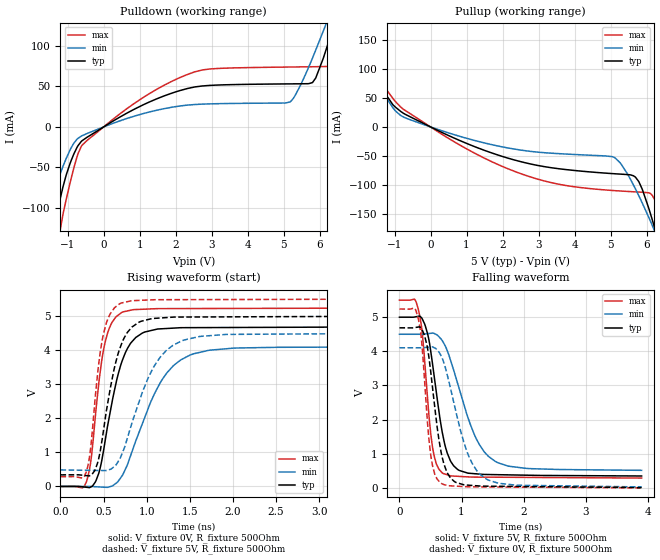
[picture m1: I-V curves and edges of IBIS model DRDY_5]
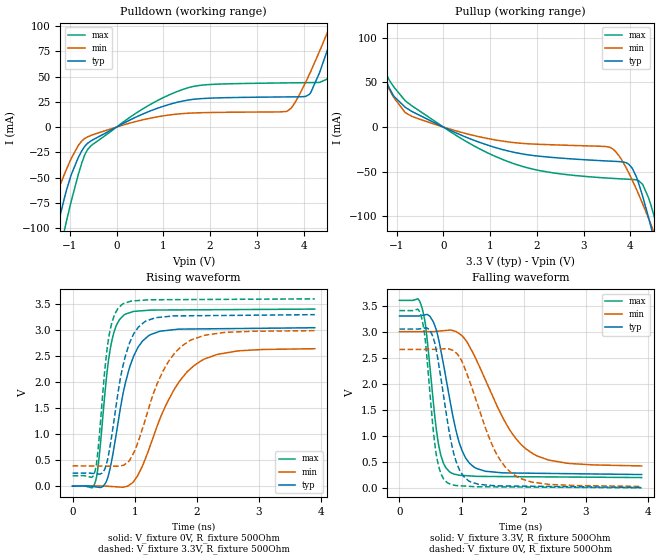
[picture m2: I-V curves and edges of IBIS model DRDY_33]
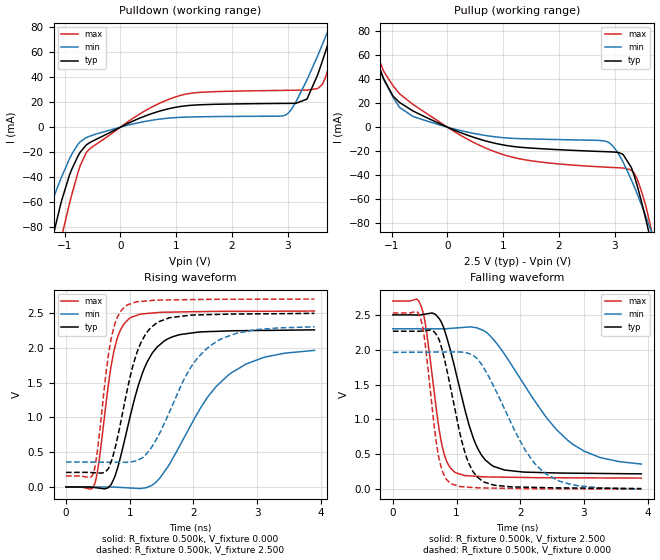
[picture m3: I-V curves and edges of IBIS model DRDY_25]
| Texas Instruments Incorporated
| Marketing part#   Voltage Range   Package-type   #pins/pkg drawing
| ADS1220PW   2.3V - 5.5V   TSSOP   16/PW
| ADS1220RVA   2.3V - 5.5V   QFN   16/RVA
| ADS1120PW   2.3V - 5.5V   TSSOP   16/PW
| ADS1120RVA   2.3V - 5.5V   QFN   16/RVA
[IBIS Ver]   4.0
[File name]   ads1220.ibs
[File Rev]   1.1
[Date]   1/15/2014
[Source]   Model built from TISpice simulations at:
   Texas Instruments Incorporated.
   Webench Design Center
   12500 TI Blvd
   Dallas, TX -75243
   For Support e-mail: elab_ibis@list.ti.com
[Notes]   Revision History
   1.1: 01/15/2014
   - Add device ADS1120PW and ADS1120RVA to supported devices
   and change name of components to represent both devices with 'x.'
   1.0   | Initial Release
   - C_comp although listed in numerical order of value are
   obtained from varying PVT conditions. For PVT conditions
   for each specific value refer the buffer description under
   respective [Model]. IBIS model user is responsible for using
   appropriate C_comp to simulate for Signal Integrity.
[Disclaimer]  This model is designed as an aid for customers of Texas Instruments
 TI and its licensors and suppliers make no warranties, either expressed
 or implied, with respect to this  model, including the warranties of
 merchantability or fitness for a particular purpose.
 The model is provided solely on an "as is" basis. The entire risk as to
 its quality and performance is with the customer.
[Copyright] (C)Copyright 2014 Texas Instruments Incorporated.
   All rights reserved.
[Component]  ADS1x20PW
[Manufacturer]  Texas Instruments
[Package]
|   typ   min   max
R_pkg   0   0   0
L_pkg   0   0   0
C_pkg   0   0   0
[Pin]   signal_name   model_name   R_pin   L_pin   C_pin
1   CLK   DIN   0.19322  2.91462n  0.47845p
2   DGND   GND   0.19290  2.48827n  0.48118p
3   AVSS   GND   0.16877  1.95590n  0.35342p
4   AIN3   TERM   0.16849  1.94998n  0.36106p
5   AIN2   TERM   0.06398  1.50548n  0.40584p
6   REFN0   TERM   0.16819  1.95272n  0.35310p
7   REFP0   TERM   0.20145  2.55201n  0.48267p
8   AIN1   TERM   0.19504  2.93239n  0.47960p
9   AIN0   TERM   0.19504  2.93239n  0.47958p
10   AVDD   POWER   0.20145  2.55201n  0.48241p
11   DVDD   POWER   0.17165  1.97913n  0.35356p
12   DRDY   DRDY   0.09379  1.65190n  0.39123p
13   DOUT   DOUT   0.16644  1.93419n  0.36060p
14   DIN   DIN   0.16865  1.95507n  0.35303p
15   SCLK   DIN   0.19362  2.49377n  0.48147p
16   CS   DIN   0.19322  2.91462n  0.47846p
[Component]  ADS1x20RVA
[Manufacturer]  Texas Instruments
[Package]
|   typ   min   max
R_pkg   0   0   0
L_pkg   0   0   0
C_pkg   0   0   0
[Pin]   signal_name   model_name   R_pin   L_pin   C_pin
1   CLK   DIN   0.06026  0.73141n  0.13625pF
2   DGND   GND   0.06340  0.77403n  0.15300pF
3   AVSS   GND   0.02077  0.40544n  0.18775pF
4   AIN3   TERM   0.06028  0.73169n  0.13612pF
5   AIN2   TERM   0.06127  0.74279n  0.13670pF
6   REFN0   TERM   0.06032  0.72840n  0.14946pF
7   REFP0   TERM   0.06032  0.72772n  0.14944pF
8   AIN1   TERM   0.06127  0.74046n  0.13654pF
9   AIN0   TERM   0.06051  0.72727n  0.13563pF
10   AVDD   POWER   0.03224  0.51093n  0.17648pF
11   DVDD   POWER   0.06123  0.73664n  0.15089pF
12   DRDY   DRDY   0.06048  0.72677n  0.13587pF
13   DOUT   DOUT   0.06057  0.73159n  0.13595pF
14   DIN   DIN   0.06026  0.72711n  0.14916pF
15   SCLK   DIN   0.06026  0.72728n  0.14916pF
16   CS   DIN   0.06037  0.72972n  0.13575pF
[Model Selector]  DIN
DIN_5   5.0V non-modeled pin
DIN_33   3.3V non-modeled pin
DIN_25   2.5V non-modeled pin
[Model Selector]  DRDY
DRDY_5   5.0V non-modeled pin
DRDY_33   3.3V non-modeled pin
DRDY_25   2.5V non-modeled pin
[Model Selector]  DOUT
DOUT_5   5.0V non-modeled pin
DOUT_33   3.3V non-modeled pin
DOUT_25   2.5V non-modeled pin
[Model Selector]  TERM
TERM_5   5.0V non-modeled pin
TERM_33   3.3V non-modeled pin
TERM_25   2.5V non-modeled pin
|   TERM Model
[Model] TERM_33
Model_type Terminator
C_comp   1e-20   1e-20   1e-20
| variable   typ   min   max
[Voltage Range]   3.3V   3.15V   3.45V
[POWER Clamp Reference]  3.3V   3.15V   3.45V
|Operating Temperature
[Temperature Range]   27   125   -40
[Model] TERM_25
Model_type Terminator
C_comp   1e-20   1e-20   1e-20
| variable   typ   min   max
[Voltage Range]   2.5V   2.375V   2.625V
[POWER Clamp Reference]  2.5V   2.375V   2.625V
[GND Clamp Reference]   0.0V   0.0V   0.0V
|Operating Temperature
[Temperature Range]   27   125   -40
[Model] TERM_5
Model_type Terminator
C_comp   1e-20   1e-20   1e-20
| variable   typ   min   max
[Voltage Range]   5.0V   4.5V   5.5V
[POWER Clamp Reference]  5.0V   4.5V   5.5V
[GND Clamp Reference]   0.0V   0.0V   0.0V
|Operating Temperature
[Temperature Range]   27   125   -40
| Models and submodels in the file (12): DRDY_5 (Output), DRDY_33 (Output), DRDY_25 (Output), DOUT_5 (3-state), DOUT_33 (3-state), DOUT_25 (3-state), DIN_5 (Input), DIN_33 (Input), DIN_25 (Input), TERM_33 (Terminator), TERM_25 (Terminator), TERM_5 (Terminator)
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|   DRDY_5 Model
[Model]   DRDY_5
Model_type   Output
Polarity   Non-Inverting
Vmeas = 2.5
Vref = 2.5
Cref = 15pF
Rref = 500
|   typ   min   max
|   (nom PVT)   (Fast PVT)   (slow PVT)
C_comp   2.792p   2.372p   3.227p
|C_comp (ON state)   2.957p   2.508p   3.404p
|C_comp (OFF state)   2.792p   2.372p   3.227p
| Where   nom PVT is  Nominal Process, 5V, 27C
|   Fast PVT is Strong Process, 5.5V, -40C
|   Slow PVT is Weak Process, 4.5V, 125C
[Voltage Range]   5   4.5   5.5
[Temperature Range]   27   125   -40
[Pullup Reference]   5   4.5   5.5
[Pulldown Reference]   0   0   0
[Power Clamp Reference]   5   4.5   5.5
[GND Clamp Reference]   0   0   0
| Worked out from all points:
|   slope of the pulldown table from 0 to 0.75 V, typ, clamps not added: 38.5 ohm
|   slope of the pullup table from 0 to 0.75 V, typ, clamps not added: 34.6 ohm
|   falling waveform, V_fixture 5V, R_fixture 500Ohm: 20-80 % time 231ps typ, 445ps min, 150ps max; typ from 5 V to 0.349 V
|   rising waveform, V_fixture 0V, R_fixture 500Ohm: 20-80 % time 233ps typ, 416ps min, 148ps max; typ from 0 V to 4.68 V
|   rising waveform, V_fixture 5V, R_fixture 500Ohm: 20-80 % time 214ps typ, 369ps min, 139ps max; typ from 0.34 V to 5 V
|   falling waveform, V_fixture 0V, R_fixture 500Ohm: 20-80 % time 203ps typ, 366ps min, 136ps max; typ from 4.69 V to 0.009 V
[Pulldown]
|   Voltage   I(typ)   I(min)   I(max)
-5V       -984.7mA   -666.3mA   -1.34A
-1.835V   -225.5mA   -142.5mA   -320.3mA
-1.52V    -154.3mA   -97.92mA   -220.6mA
-1.25V    -96.93mA   -62.99mA   -138.7mA
-605mV    -17.19mA   -11mA      -22.85mA
2.32V     47.36mA    26.92mA    64.68mA
5.17V     53.16mA    30.73mA    73.97mA
5.8V      54.77mA    84.97mA    74.32mA
6.25V     105.4mA    135.3mA    74.76mA
6.415V    129.1mA    154.2mA    79.06mA
7.09V     229.8mA    232.8mA    195.3mA
10V       695.5mA    589.2mA    793.5mA
[Pullup]
|   Voltage   I(typ)   I(min)   I(max)
-5V       615.3mA    484.3mA    781.6mA
-2.36V    216.2mA    176.1mA    268.1mA
-2.195V   191.6mA    157.1mA    236.3mA
-1.97V    158.2mA    131.4mA    193.3mA
-965mV    33.47mA    26.93mA    42.93mA
820mV     -23.56mA   -16.29mA   -31.34mA
2.95V     -65.85mA   -43.15mA   -89.22mA
5.095V    -80.35mA   -52.09mA   -109.3mA
5.695V    -86.53mA   -106.8mA   -111.6mA
6.25V     -178.5mA   -182.4mA   -127.7mA
6.49V     -231.1mA   -218.4mA   -172.3mA
10V       -1.077A    -812.1mA   -1.299A
[Ramp]
R_load = 500
|   typ   min   max
dV/dt_r   2.81122/2.31953e-10   2.45779/4.13764e-10   3.14302/1.47295e-10
dV/dt_f   2.79077/2.30674e-10   2.39144/4.43892e-10   3.12731/1.49622e-10
[Falling Waveform]
V_fixture = 5V
V_fixture_min = 4.5V
V_fixture_max = 5.5V
R_fixture = 500Ohm
C_fixture = 0F
|   Time   V(typ)   V(min)   V(max)
0s        5V         4.5V       5.5V
301.3ps   5.024V     4.5V       5.249V
371.3ps   4.936V     4.502V     4.473V
529ps     3.685V     4.532V     1.238V
685.9ps   1.663V     4.323V     444.6mV
769.3ps   1.022V     4.02V      383.9mV
935.2ps   542.4mV    3.072V     340.2mV
1.236ns   412mV      1.445V     316.7mV
1.544ns   388.3mV    775.6mV    313.3mV
3.9ns     348.7mV    514.3mV    287.8mV
[Rising Waveform]
V_fixture = 0V
V_fixture_min = 0V
V_fixture_max = 0V
R_fixture = 500Ohm
C_fixture = 0F
|   Time   V(typ)   V(min)   V(max)
0s        4.594nV    7.392nV    3.899nV
301.3ps   -24.2mV    1.124mV    139.9mV
356.5ps   -8.175mV   -908.9uV   823.3mV
413.5ps   178.3mV    -9.035mV   2.296V
505.6ps   1.141V     -22.14mV   4.09V
706.2ps   3.619V     283.1mV    5.102V
873.5ps   4.375V     1.338V     5.194V
1.154ns   4.626V     3.031V     5.221V
1.5ns     4.662V     3.854V     5.223V
3.9ns     4.685V     4.096V     5.238V
[Rising Waveform]
V_fixture = 5V
V_fixture_min = 4.5V
V_fixture_max = 5.5V
R_fixture = 500Ohm
C_fixture = 0F
|   Time   V(typ)   V(min)   V(max)
0s        340.2mV    485.1mV    286.7mV
297.8ps   318.2mV    474.7mV    416.5mV
347ps     325.1mV    472.9mV    1.061V
404.3ps   504.9mV    470.9mV    2.651V
490.1ps   1.488V     467.9mV    4.375V
685.9ps   4.033V     801.1mV    5.363V
829.5ps   4.681V     1.868V     5.454V
1.064ns   4.93V      3.427V     5.479V
1.397ns   4.974V     4.265V     5.485V
3.9ns     4.998V     4.494V     5.5V
[Falling Waveform]
|Gnd
V_fixture = 0V
V_fixture_min = 0V
V_fixture_max = 0V
R_fixture = 500Ohm
C_fixture = 0F
|   Time   V(typ)   V(min)   V(max)
0s        4.688V     4.104V     5.239V
297.8ps   4.711V     4.103V     4.998V
362.6ps   4.642V     4.106V     4.19V
499.9ps   3.458V     4.126V     1.018V
565.1ps   2.423V     4.1V       425.1mV
658.7ps   1.172V     3.912V     150.9mV
819ps     296.5mV    2.942V     59.86mV
1.091ns   81.82mV    1.045V     34.35mV
1.397ns   50.88mV    262.5mV    28.41mV
3.9ns     8.998mV    28.15mV    1.283mV
|   DRDY_33 Model
[Model]   DRDY_33
Model_type   Output
Polarity   Non-Inverting
Vmeas = 1.65
Vref = 1.65
Cref = 15pF
Rref = 500
|   typ   min   max
|   (nom PVT)   (Fast PVT)   (slow PVT)
C_comp   3.004p   2.545p   3.470p
|C_comp (ON state)   3.156p   2.689p   3.615p
|C_comp (OFF state)   3.004p   2.545p   3.470p
| Where   nom PVT is  Nominal Process, 3.3V, 27C
|   Fast PVT is Strong Process, 3.6V, -40C
|   Slow PVT is Weak Process, 3.0V, 125C
[Voltage Range]   3.3   3   3.6
[Temperature Range]   27   125   -40
[Pullup Reference]   3.3   3   3.6
[Pulldown Reference]   0   0   0
[Power Clamp Reference]   3.3   3   3.6
[GND Clamp Reference]   0   0   0
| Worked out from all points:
|   slope of the pulldown table from 0 to 0.495 V, typ, clamps not added: 42.9 ohm
|   slope of the pullup table from 0 to 0.495 V, typ, clamps not added: 42.9 ohm
|   falling waveform, V_fixture 3.3V, R_fixture 500Ohm: 20-80 % time 306ps typ, 654ps min, 183ps max; typ from 3.3 V to 0.256 V
|   rising waveform, V_fixture 0V, R_fixture 500Ohm: 20-80 % time 316ps typ, 614ps min, 182ps max; typ from 0 V to 3.04 V
|   rising waveform, V_fixture 3.3V, R_fixture 500Ohm: 20-80 % time 283ps typ, 517ps min, 168ps max; typ from 0.248 V to 3.3 V
|   falling waveform, V_fixture 0V, R_fixture 500Ohm: 20-80 % time 261ps typ, 507ps min, 163ps max; typ from 3.05 V to 0.008 V
[Pulldown]
|   Voltage   I(typ)   I(min)   I(max)
-3.3V     -573.5mA   -376.1mA   -791.3mA
-1.736V   -202.6mA   -128mA     -288.6mA
-1.3V     -106.7mA   -68.95mA   -152.7mA
-1.112V   -69.7mA    -46.43mA   -101.8mA
-617.1mV  -16mA      -9.682mA   -22.14mA
709.5mV   15.75mA    8.689mA    22.07mA
1.68V     27.68mA    14.03mA    40.59mA
3.64V     29.87mA    15.63mA    43.78mA
4.135V    32.91mA    53.13mA    44.04mA
4.561V    83.38mA    99.24mA    52.5mA
4.957V    140.9mA    144.3mA    119.8mA
6.6V      389.2mA    336mA      438.2mA
[Pullup]
|   Voltage   I(typ)   I(min)   I(max)
-3.3V     357.5mA    285.1mA    450.1mA
-1.934V   152.6mA    127mA      186.1mA
-1.399V   75.08mA    67.22mA    86.57mA
-1.053V   34.09mA    32.4mA     44.39mA
-636.9mV  16.5mA     11.25mA    22.48mA
1.403V    -27.01mA   -16.73mA   -39.08mA
3.571V    -38.19mA   -22.89mA   -57.36mA
4.046V    -46.68mA   -60.1mA    -58.74mA
4.264V    -77.65mA   -86.15mA   -64.23mA
4.442V    -112mA     -109.4mA   -87.85mA
4.58V     -141mA     -128.5mA   -116mA
6.6V      -616.6mA   -451.2mA   -757.4mA
[Ramp]
R_load = 500
|   typ   min   max
dV/dt_r   1.82672/3.14339e-10   1.58478/6.10418e-10   2.04187/1.81599e-10
dV/dt_f   1.82616/3.05643e-10   1.54681/6.52787e-10   2.04071/1.8322e-10
[Falling Waveform]
V_fixture = 3.3V
V_fixture_min = 3V
V_fixture_max = 3.6V
R_fixture = 500Ohm
C_fixture = 0F
|   Time   V(typ)   V(min)   V(max)
0s        3.3V       3V         3.6V
357.9ps   3.31V      3V         3.479V
431ps     3.327V     3V         3.017V
622.4ps   2.897V     3.008V     885.9mV
804.8ps   1.736V     3.028V     311.6mV
960.8ps   877.3mV    2.962V     244mV
1.128ns   474.3mV    2.715V     230.9mV
1.664ns   288.6mV    1.348V     217.5mV
2.039ns   283.1mV    746.2mV    214.4mV
3.9ns     256.4mV    422mV      198.8mV
[Rising Waveform]
V_fixture = 0V
V_fixture_min = 0V
V_fixture_max = 0V
R_fixture = 500Ohm
C_fixture = 0F
|   Time   V(typ)   V(min)   V(max)
0s        3.316nV    5.881nV    2.676nV
367.3ps   -14.29mV   506.1uV    80.56mV
494.2ps   -4.617mV   681.1uV    1.424V
606.1ps   347.8mV    -7.027mV   2.631V
827.6ps   1.86V      -19.73mV   3.289V
984.1ps   2.5V       89.37mV    3.359V
1.222ns   2.888V     679.6mV    3.381V
1.618ns   3.006V     1.818V     3.387V
1.953ns   3.021V     2.314V     3.389V
3.9ns     3.045V     2.641V     3.403V
[Rising Waveform]
V_fixture = 3.3V
V_fixture_min = 3V
V_fixture_max = 3.6V
R_fixture = 500Ohm
C_fixture = 0F
|   Time   V(typ)   V(min)   V(max)
0s        247.9mV    388.3mV    197.7mV
357.9ps   238.3mV    384.7mV    267.2mV
407.5ps   232.1mV    384.2mV    658.8mV
476.3ps   249mV      383.5mV    1.633V
579.2ps   600.8mV    382.5mV    2.83V
794.1ps   2.216V     393.2mV    3.491V
1.059ns   3.055V     864.3mV    3.567V
1.368ns   3.241V     1.982V     3.583V
1.755ns   3.273V     2.689V     3.586V
3.9ns     3.296V     2.988V     3.6V
[Falling Waveform]
|Gnd
V_fixture = 0V
V_fixture_min = 0V
V_fixture_max = 0V
R_fixture = 500Ohm
C_fixture = 0F
|   Time   V(typ)   V(min)   V(max)
0s        3.049V     2.657V     3.404V
349.4ps   3.057V     2.657V     3.298V
416.1ps   3.07V      2.657V     2.836V
590.1ps   2.662V     2.662V     664.9mV
764.2ps   1.35V      2.671V     106.9mV
887.5ps   602.7mV    2.615V     51.12mV
1.033ns   220.7mV    2.354V     36.54mV
1.459ns   49.08mV    919.8mV    20.83mV
1.802ns   35.91mV    288.1mV    18.07mV
3.9ns     8.283mV    28.1mV     1.174mV
|   DRDY_25 Model
[Model]   DRDY_25
Model_type   Output
Polarity   Non-Inverting
Vmeas = 1.25
Vref = 1.25
Cref = 15pF
Rref = 500
|   typ   min   max
|   (nom PVT)   (Fast PVT)   (slow PVT)
C_comp   3.118p   2.644p   3.607p
|C_comp (ON state)   3.233p   2.765p   3.707p
|C_comp (OFF state)   3.118p   2.644p   3.607p
| Where   nom PVT is  Nominal Process, 2.5V, 27C
|   Fast PVT is Strong Process, 2.7V, -40C
|   Slow PVT is Weak Process, 2.3V, 125C
[Voltage Range]   2.5   2.3   2.7
[Temperature Range]   27   125   -40
[Pullup Reference]   2.5   2.3   2.7
[Pulldown Reference]   0   0   0
[Power Clamp Reference]   2.5   2.3   2.7
[GND Clamp Reference]   0   0   0
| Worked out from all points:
|   slope of the pulldown table from 0 to 0.375 V, typ, clamps not added: 48.5 ohm
|   slope of the pullup table from 0 to 0.375 V, typ, clamps not added: 54 ohm
|   falling waveform, R_fixture 0.500k, V_fixture 2.500: 20-80 % time 399ps typ, 920ps min, 224ps max; typ from 2.5 V to 0.219 V
|   rising waveform, R_fixture 0.500k, V_fixture 0.000: 20-80 % time 419ps typ, 839ps min, 234ps max; typ from 0 V to 2.26 V
|   rising waveform, R_fixture 0.500k, V_fixture 2.500: 20-80 % time 362ps typ, 670ps min, 211ps max; typ from 0.21 V to 2.49 V
|   falling waveform, R_fixture 0.500k, V_fixture 0.000: 20-80 % time 332ps typ, 676ps min, 195ps max; typ from 2.27 V to 0.009 V
[Pulldown]
|   Voltage   I(typ)   I(min)   I(max)
-2.5V     -381.6mA   -244.9mA   -533.5mA
-1.562V   -163.3mA   -103.5mA   -233.5mA
-1.173V   -80.44mA   -53.2mA    -115.3mA
-1.06V    -59.61mA   -40.37mA   -88.71mA
-865mV    -32.97mA   -21.12mA   -52.82mA
-617.5mV  -14.49mA   -8.471mA   -20.69mA
1.04V     16.32mA    7.778mA    24.99mA
2.953V    19.03mA    9.601mA    29.47mA
3.342V    22.46mA    37.81mA    29.68mA
3.703V    64.32mA    75.35mA    43.49mA
4.07V     117.2mA    116.7mA    107.9mA
5V        256.1mA    224mA      286.2mA
[Pullup]
|   Voltage   I(typ)   I(min)   I(max)
-2.5V     236.9mA    192.1mA    294.8mA
-1.577V   100.1mA    86.64mA    118.5mA
-970mV    25.73mA    24.64mA    34.34mA
-617.5mV  13.51mA    8.979mA    19mA
327.5mV   -6.164mA   -3.813mA   -9.218mA
957.5mV   -14.48mA   -8.605mA   -22.28mA
2.848V    -20.51mA   -11.87mA   -33.44mA
3.155V    -23.15mA   -29.63mA   -34.16mA
3.35V     -40.59mA   -49.72mA   -38.48mA
3.56V     -77.34mA   -74.75mA   -66.1mA
3.665V    -98.3mA    -88.2mA    -87.32mA
5V        -404.4mA   -289.4mA   -505.7mA
[Ramp]
R_load = 500
|   typ   min   max
dV/dt_r   1.35427/4.18079e-10   1.1489/8.34099e-10   1.51596/2.32215e-10
dV/dt_f   1.36834/3.99329e-10   1.12494/9.13308e-10   1.52458/2.23866e-10
[Falling Waveform]
R_fixture = 0.500k
V_fixture = 2.500
V_fixture_min = 2.300
V_fixture_max = 2.700
C_fixture = 0.000
|  time   V(typ)   V(min)   V(max)
0s        2.5V       2.3V       2.7V
449.7ps   2.502V     2.3V       2.611V
524.3ps   2.514V     2.3V       2.288V
759ps     2.399V     2.3V       685mV
847.3ps   2.174V     2.302V     394.9mV
964.9ps   1.769V     2.31V      248.9mV
1.274ns   705.5mV    2.321V     186.2mV
1.565ns   335.8mV    2.162V     174.8mV
2.748ns   229.9mV    697.6mV    162.9mV
3.9ns     219.4mV    360.1mV    159mV
[Rising Waveform]
R_fixture = 0.500k
V_fixture = 0.000
V_fixture_min = 0.000
V_fixture_max = 0.000
C_fixture = 0.000
|  time   V(typ)   V(min)   V(max)
0s        2.773nV    -87.82nV   2.124nV
447ps     -6.979mV   300.2uV    35.77mV
517ps     -15.21mV   347.2uV    358.1mV
742.4ps   99.78mV    324uV      1.905V
990.8ps   948.3mV    -12.62mV   2.418V
1.274ns   1.795V     -4.691mV   2.492V
1.607ns   2.131V     303mV      2.511V
2.208ns   2.231V     1.27V      2.52V
2.565ns   2.242V     1.618V     2.523V
3.9ns     2.257V     1.962V     2.527V
[Rising Waveform]
R_fixture = 0.500k
V_fixture = 2.500
V_fixture_min = 2.300
V_fixture_max = 2.700
C_fixture = 0.000
|  time   V(typ)   V(min)   V(max)
0s        209.9mV    360.1mV    157.8mV
428.9ps   206.5mV    357.9mV    192.6mV
497.3ps   203mV      357.5mV    543.2mV
706.8ps   358.9mV    356.5mV    2.115V
940.8ps   1.303V     355.3mV    2.601V
1.175ns   2.07V      408.4mV    2.665V
1.453ns   2.372V     742.2mV    2.684V
1.95ns    2.467V     1.704V     2.691V
2.297ns   2.477V     2.049V     2.695V
3.9ns     2.494V     2.3V       2.699V
[Falling Waveform]
R_fixture = 0.500k
V_fixture = 0.000
V_fixture_min = 0.000
V_fixture_max = 0.000
C_fixture = 0.000
|  time   V(typ)   V(min)   V(max)
0s        2.266V     1.962V     2.527V
433.4ps   2.267V     1.965V     2.454V
503.6ps   2.274V     1.965V     2.115V
706.8ps   2.181V     1.967V     527mV
896.8ps   1.497V     1.968V     88.81mV
1.146ns   482.9mV    1.958V     31.05mV
1.418ns   109.3mV    1.753V     17.72mV
2.056ns   29.01mV    593.4mV    9.137mV
2.386ns   22.15mV    231.4mV    6.039mV
3.9ns     8.55mV     -87.82nV   1.176mV
